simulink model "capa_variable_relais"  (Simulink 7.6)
settings: Solver=ode15s  StartTime=0.0  StopTime=N  RelTol=1e-3
InitFcn:
  | N=450;
StopFcn:
  | clc, close all
  | load sortie_RC.mat
  | plot(x(1,:), x(2,:),x(1,:), x(3,:),x(1,:), x(4,:))
  | grid
  | title('Charge et décharge d''une capacité variable')
  | xlabel('temps')
  | axis([0 450 -0.2 2.2])
undefined symbols (not defined in the file or in its folder): sigbuilder_block
libraries: fl_lib x11, nesl_utility x5, simulink x1

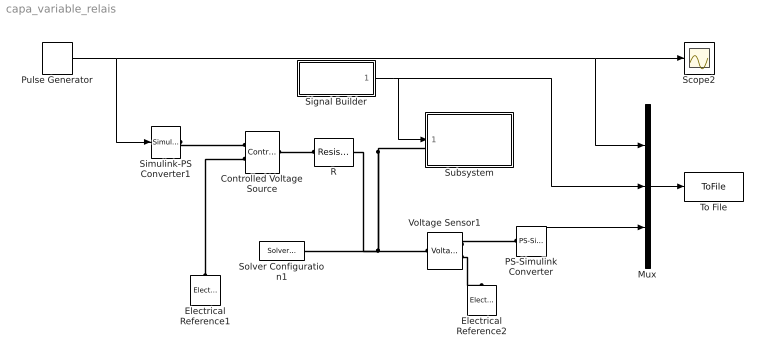
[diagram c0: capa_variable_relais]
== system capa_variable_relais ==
  Controlled Voltage Source : fl_lib/Electrical/Electrical Sources/Controlled Voltage Source  DialogController=NetworkEngine.DynNeDlgSource  SystemSampleTime=-1  i_Log=off  v_Log=off  LocalVarNames=|current|voltage|power  LocalVarDescs=|Current (A)|Voltage (V)|Power (W)  LocalVarLogging=[0 0 0]
  Electrical Reference1 : fl_lib/Electrical/Electrical Elements/Electrical Reference  DialogController=NetworkEngine.DynNeDlgSource  SystemSampleTime=-1  i_Log=off  LocalVarNames=|i  LocalVarDescs=|i  LocalVarLogging=0
  Electrical Reference2 : fl_lib/Electrical/Electrical Elements/Electrical Reference  DialogController=NetworkEngine.DynNeDlgSource  SystemSampleTime=-1  i_Log=off  LocalVarNames=|i  LocalVarDescs=|i  LocalVarLogging=0
  Mux : Mux  Inputs=3
  PS-Simulink Converter : nesl_utility/PS-Simulink Converter  DialogController=NetworkEngine.DynNeUtilDlgSource  SystemSampleTime=-1  PhysicalDomain=network_engine_domain  LeftPortType=input  RightPortType=output  SubClassName=ps_output  Unit=1  AffineConversion=off
  Pulse Generator : DiscretePulseGenerator  PulseType=Time based  Amplitude=2  Period=250  PulseWidth=50
  R : fl_lib/Electrical/Electrical Elements/Resistor  DialogController=NetworkEngine.DynNeDlgSource  SystemSampleTime=-1  R=1 kOhm  i_Log=off  v_Log=off  LocalVarNames=|i|v  LocalVarDescs=|i|v  LocalVarLogging=[0 0]
  Scope2 : Scope
  Signal Builder : Subsystem  Tag=STV Subsys  LoadFcn=sigbuilder_block('load');  StartFcn=sigbuilder_block('start');  StopFcn=sigbuilder_block('stop');  ClipboardFcn=sigbuilder_block('clipboard');
  Simulink-PS Converter1 : nesl_utility/Simulink-PS Converter  DialogController=NetworkEngine.DynNeUtilDlgSource  SystemSampleTime=-1  PhysicalDomain=network_engine_domain  LeftPortType=input  RightPortType=output  SubClassName=ps_input  Unit=1  AffineConversion=off  InputFilterTimeConstant=.001  UdotUserProvided=0
  Solver Configuration1 : nesl_utility/Solver Configuration  DialogController=NetworkEngine.DynNeUtilDlgSource  SystemSampleTime=-1  PhysicalDomain=network_engine_domain  LeftPortType=input  RightPortType=generic  SubClassName=solver  Accelerate=off  Profile=off  ResidualTolerance=1e-9  MaxNonlinIter=12  MaxModeIter=2  DoFixedCost=off  UseLocalSampling=off  DoDC=off  LinearAlgebra=Sparse  LocalSolverSampleTime=.001  LocalSolverChoice=NE_BACKWARD_EULER_ADVANCER  UseLocalSolver=off
  Subsystem : Subsystem
  To File : ToFile  Filename=sortie_RC  MatrixName=x
  Voltage Sensor1 : fl_lib/Electrical/Electrical Sensors/Voltage Sensor  DialogController=NetworkEngine.DynNeDlgSource  SystemSampleTime=-1  i1_Log=off  v1_Log=off  LocalVarNames=|i1|v1  LocalVarDescs=|i1|v1  LocalVarLogging=[0 0]
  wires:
  Pulse Generator/1 -> Simulink-PS Converter1/1, Scope2/1, Mux/1
  Signal Builder/1(Signal 2) -> Subsystem/1(capa), Mux/2
  Mux/1 -> To File/1
  PS-Simulink Converter/1 -> Mux/3
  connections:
  R/RConn1 -- Subsystem/LConn1 -- Voltage Sensor1/LConn1 -- Solver Configuration1/RConn1
  Simulink-PS Converter1/RConn1 -- Controlled Voltage Source/RConn1
  Electrical Reference1/LConn1 -- Controlled Voltage Source/RConn2
  Controlled Voltage Source/LConn1 -- R/LConn1
  Voltage Sensor1/RConn1 -- PS-Simulink Converter/LConn1
  Voltage Sensor1/RConn2 -- Electrical Reference2/LConn1

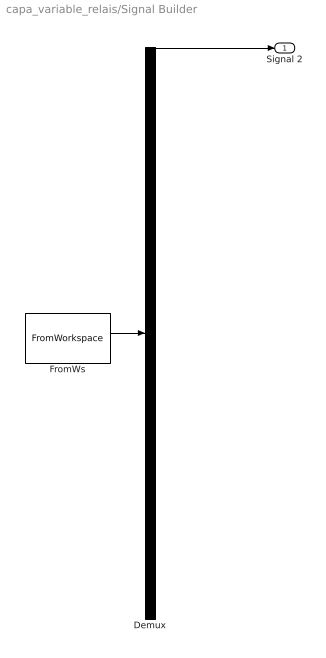
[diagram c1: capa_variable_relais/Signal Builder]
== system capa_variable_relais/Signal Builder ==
  Demux : Demux  Tag=STV Demux  Outputs=1
  FromWs : FromWorkspace  Tag=STV FromWs  VariableName=tuvar  SampleTime=0  SigBuilderData=DataTag0  VnvData=DataTag1
  Signal 2 : Outport  Tag=STV Outport
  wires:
  FromWs/1 -> Demux/1
  Demux/1 -> Signal 2/1

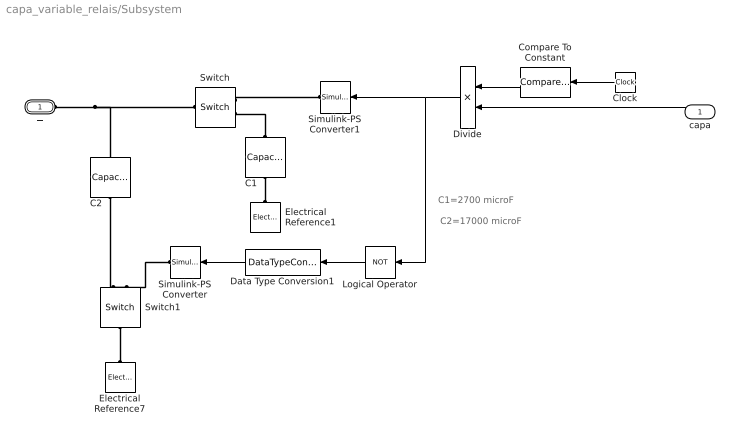
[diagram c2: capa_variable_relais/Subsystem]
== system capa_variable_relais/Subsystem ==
  note: C1=2700 microF
  note: C2=17000 microF
  capa : Inport
  C1 : fl_lib/Electrical/Electrical Elements/Capacitor  DialogController=NetworkEngine.DynNeDlgSource  SystemSampleTime=-1  c=2700 uF  v0=0 V  r=1e-9 Ohm  g=0 1/Ohm  i_Log=off  v_Log=off  vc_Log=off  LocalVarNames=|i|v|vc  LocalVarDescs=|i|v|Internal variable for voltage across capacitor term  LocalVarLogging=[0 0 0]
  C2 : fl_lib/Electrical/Electrical Elements/Capacitor  DialogController=NetworkEngine.DynNeDlgSource  SystemSampleTime=-1  c=17000 uF  v0=0 V  r=1e-9 Ohm  g=0 1/Ohm  i_Log=off  v_Log=off  vc_Log=off  LocalVarNames=|i|v|vc  LocalVarDescs=|i|v|Internal variable for voltage across capacitor term  LocalVarLogging=[0 0 0]
  Clock : Clock
  Compare To Constant : simulink/Logic and Bit Operations/Compare To Constant  SystemSampleTime=-1  relop=<=  const=250  LogicOutDataTypeMode=uint8
  Data Type Conversion1 : DataTypeConversion  OutDataTypeStr=double
  Divide : Product  Inputs=**
  Electrical Reference1 : fl_lib/Electrical/Electrical Elements/Electrical Reference  DialogController=NetworkEngine.DynNeDlgSource  SystemSampleTime=-1  i_Log=off  LocalVarNames=|i  LocalVarDescs=|i  LocalVarLogging=0
  Electrical Reference7 : fl_lib/Electrical/Electrical Elements/Electrical Reference  DialogController=NetworkEngine.DynNeDlgSource  SystemSampleTime=-1  i_Log=off  LocalVarNames=|i  LocalVarDescs=|i  LocalVarLogging=0
  Logical Operator : Logic  Operator=NOT  AllPortsSameDT=off  OutDataTypeStr=boolean
  Simulink-PS Converter : nesl_utility/Simulink-PS Converter  DialogController=NetworkEngine.DynNeUtilDlgSource  SystemSampleTime=-1  PhysicalDomain=network_engine_domain  LeftPortType=input  RightPortType=output  SubClassName=ps_input  Unit=1  AffineConversion=off  InputFilterTimeConstant=.001  UdotUserProvided=0
  Simulink-PS Converter1 : nesl_utility/Simulink-PS Converter  DialogController=NetworkEngine.DynNeUtilDlgSource  SystemSampleTime=-1  PhysicalDomain=network_engine_domain  LeftPortType=input  RightPortType=output  SubClassName=ps_input  Unit=1  AffineConversion=off  InputFilterTimeConstant=.001  UdotUserProvided=0
  Switch : fl_lib/Electrical/Electrical Elements/Switch  DialogController=NetworkEngine.DynNeDlgSource  SystemSampleTime=-1  R_closed=0.001 Ohm  G_open=1e-10 1/Ohm  Threshold=0.5  i_Log=off  v_Log=off  LocalVarNames=|i|v  LocalVarDescs=|i|v  LocalVarLogging=[0 0]
  Switch1 : fl_lib/Electrical/Electrical Elements/Switch  DialogController=NetworkEngine.DynNeDlgSource  SystemSampleTime=-1  R_closed=0.001 Ohm  G_open=1e-10 1/Ohm  Threshold=0.5  i_Log=off  v_Log=off  LocalVarNames=|i|v  LocalVarDescs=|i|v  LocalVarLogging=[0 0]
  + : PMIOPort  Port=1  Side=Left
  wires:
  Data Type Conversion1/1 -> Simulink-PS Converter/1
  Logical Operator/1 -> Data Type Conversion1/1
  Clock/1 -> Compare To Constant/1
  Compare To Constant/1 -> Divide/1
  capa/1 -> Divide/2
  Divide/1 -> Simulink-PS Converter1/1, Logical Operator/1
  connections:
  Simulink-PS Converter/RConn1 -- Switch1/RConn1
  Switch1/LConn1 -- Electrical Reference7/LConn1
  C2/LConn1 -- Switch1/RConn2
  +/RConn1 -- C2/RConn1 -- Switch/LConn1
  Switch/RConn1 -- Simulink-PS Converter1/RConn1
  C1/RConn1 -- Switch/RConn2
  Electrical Reference1/LConn1 -- C1/LConn1
